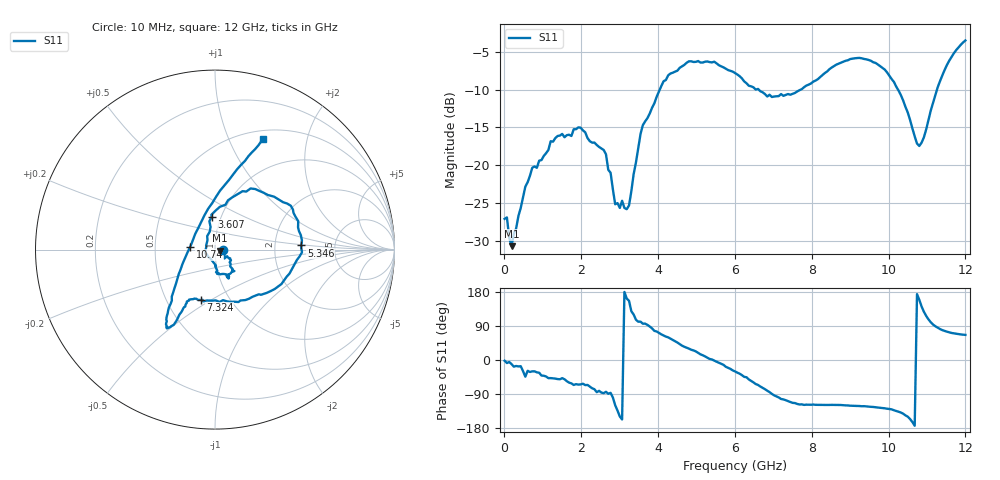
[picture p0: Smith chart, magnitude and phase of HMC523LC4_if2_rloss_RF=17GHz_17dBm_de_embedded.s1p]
!Hittite Microwave Corporation
!20 Alpha Rd
!Chelmsford, MA 01824
!Tel: 978-250-3343
!Fax: 978-250-3373
!Device: HMC523LC4, 0.01-12 GHz, GaAs MMIC Double-Balanced Mixer
!Misc: IF2 Return Loss with RF=17GHz at 17 dBm, Room
# MHZ S MA R 50
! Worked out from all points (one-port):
!   201 points, 10 MHz to 12 GHz, reference 50 ohm
!   lowest |S11| = -30.8 dB at 189.8 MHz (marker M1), VSWR 1.06, Z = 52.9 - j0.574 ohm
!   |S11| at or under -10 dB: start of sweep to 4.046 GHz; 6.625 GHz to 7.71 GHz (1.086 GHz wide, 15.1 % of centre); 10.25 GHz to 11.26 GHz (1.012 GHz wide, 9.41 % of centre)
!   S11 on the Smith chart (normalised r, x): 10 MHz: 1.09, -0.00; 3.607 GHz: 0.90, +0.34; 5.346 GHz: 2.85, +0.17; 7.324 GHz: 0.73, -0.45; 10.74 GHz: 0.76, +0.02; 12 GHz: 0.60, +1.35
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10  0.044 -2.0
69.95  0.045 -8.0
189.85  0.029 -10.8
549.55  0.072 -44.1
729.4  0.096 -29.9
1508.75  0.161 -47.9
1988.35  0.177 -64.4
2587.85  0.126 -87.5
2767.7  0.089 -86.6
2887.6  0.055 -119.5
3007.5  0.052 -149.0
3247.3  0.054 156.3
3607  0.184 95.8
4146.55  0.36 64.7
4506.25  0.423 46.1
4806  0.488 30.0
5345.55  0.482 2.7
6005  0.408 -30.1
6844.3  0.285 -81.1
7323.9  0.292 -106.0
7503.75  0.297 -113.1
9002.5  0.505 -120.6
9901.75  0.43 -127.4
10501.25  0.223 -149.6
10741.05  0.139 173.8
10920.9  0.153 127.1
11520.4  0.462 74.7
12000  0.671 66.3
